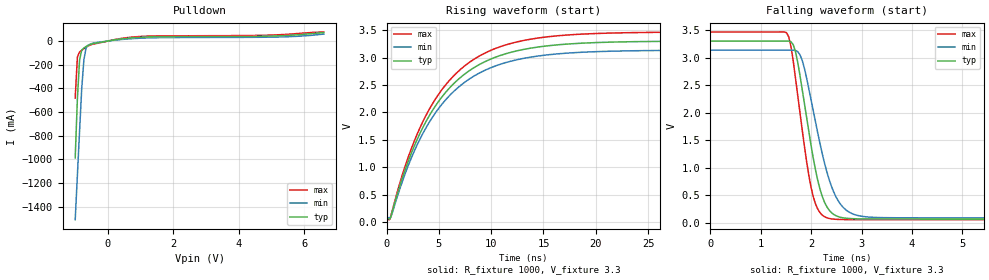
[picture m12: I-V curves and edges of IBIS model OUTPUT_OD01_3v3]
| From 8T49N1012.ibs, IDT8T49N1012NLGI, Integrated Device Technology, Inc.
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| 4.00000e+00   -1.40232e-02   -4.76240e-01   -2.57124e-03
| 4.10000e+00   -3.15805e-02   -7.57960e-01   -1.15576e-02
| 4.20000e+00   -2.28086e-01   -1.04031e+00   -2.65883e-02
| 4.30000e+00   -6.05610e-01   -1.32309e+00   -4.22837e-02
| 4.40000e+00   -9.83731e-01   -1.60621e+00   -8.93892e-02
| 4.50000e+00   -1.36238e+00   -1.88966e+00   -5.31530e-01
| 4.60000e+00   -1.74151e+00   -2.17340e+00   -1.01600e+00
| 4.70000e+00   -2.12106e+00   -2.45742e+00   -1.50101e+00
| 4.80000e+00   -2.50099e+00   -2.74170e+00   -1.98646e+00
| 4.90000e+00   -2.88126e+00   -3.02624e+00   -2.47229e+00
| 5.00000e+00   -3.26181e+00   -3.31101e+00   -2.95842e+00
| 5.10000e+00   -3.64262e+00   -3.59599e+00   -3.44478e+00
| 5.20000e+00   -4.02364e+00   -3.88118e+00   -3.93135e+00
| 5.30000e+00   -4.40484e+00   -4.16656e+00   -4.41808e+00
| 5.40000e+00   -4.78621e+00   -4.45212e+00   -4.90496e+00
| 5.50000e+00   -5.16771e+00   -4.73783e+00   -5.39197e+00
| 5.60000e+00   -5.54933e+00   -5.02369e+00   -5.87906e+00
| 5.70000e+00   -5.93104e+00   -5.30969e+00   -6.36623e+00
| 5.80000e+00   -6.31284e+00   -5.59582e+00   -6.85344e+00
| 5.90000e+00   -6.69471e+00   -5.88206e+00   -7.34069e+00
| 6.00000e+00   -7.07663e+00   -6.16842e+00   -7.82796e+00
| 6.10000e+00   -7.45860e+00   -6.45487e+00   -8.31524e+00
| 6.20000e+00   -7.84061e+00   -6.74142e+00   -8.80252e+00
| 6.30000e+00   -8.22265e+00   -7.02805e+00   -9.28980e+00
| 6.40000e+00   -8.60472e+00   -7.31476e+00   -9.77706e+00
| 6.50000e+00   -8.98680e+00   -7.60155e+00   -1.02643e+01
| 6.60000e+00   -9.36890e+00   -7.88842e+00   -1.07515e+01
[Model] OUTPUT_OD01_3v3
Model_type   Open_drain
Polarity   Non-Inverting
|   typ   min   max
C_comp   2pF   1.5pF   2.5pF
Vmeas = 1.65V
Rref = 1000
Cref = 0
Vref = 3.3V
|   typ   min   max
[Voltage range]   3.3V   3.135V   3.465V
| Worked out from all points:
|   slope of the pulldown table from 0 to 0.495 V, typ, clamps not added: 24.6 ohm
|   rising waveform, R_fixture 1000, V_fixture 3.3: 20-80 % time 5.81ns typ, 5.87ns min, 5.76ns max; typ from 0.066 V to 3.3 V
|   falling waveform, R_fixture 1000, V_fixture 3.3: 20-80 % time 364ps typ, 455ps min, 312ps max; typ from 3.3 V to 0.066 V
[Pulldown]
|Note, modeling breaks down at 250mA and above.  This is well beyond the functional   |
|operating range of the device.  Should this scenario occur, catastrophic failure and   |
|possible damage to the device and/or board is of higher concern than the I-V curve   |
|behavior.  The IBIS checker will flag currents in excess of 10A with warnings.  Lines   |
|with currents in excess of 0.35 A have been commented out.  The points still remain|
|available to the user if the user desires to use them.   |
|Voltage   I (typ)   I (min)   I (max)
|-3.30000e+00   -1.82727e+01   -1.44945e+01   -2.25188e+01
|-2.84000e+00   -1.48135e+01   -1.18930e+01   -1.81101e+01
|-2.38000e+00   -1.13544e+01   -9.29315e+00   -1.37009e+01
|-1.92000e+00   -7.89630e+00   -6.69545e+00   -9.29169e+00
|-1.46000e+00   -4.44012e+00   -4.10091e+00   -4.88327e+00
-1V       -988.4mA   -1.511A    -482.7mA
-932.9mV  -486.9mA   -1.134A    -135.3mA
-866.8mV  -160.7mA   -762.8mA   -91.83mA
-800.8mV  -75.99mA   -401.8mA   -79.06mA
-734.7mV  -58.48mA   -159.9mA   -65.71mA
-668.6mV  -46.68mA   -58.37mA   -52.4mA
-602.5mV  -36.75mA   -35.1mA    -41.15mA
-272.1mV  -13.27mA   -9.902mA   -16.62mA
388.7mV   16.58mA    12.16mA    20.94mA
983.4mV   31.27mA    23.72mA    38.36mA
5.121V    42.77mA    33.37mA    51.42mA
6.6V      70.77mA    58.76mA    76.56mA
[Ramp]
|   typ   min   max
dV/dt_r   1.942/5.814n   1.829/5.871n   2.048/5.757n
dV/dt_f   1.94/0.364n   1.829/0.455n   2.047/0.311n
R_load =   50.0000
[Rising Waveform]
R_fixture = 1000
V_fixture = 3.3
V_fixture_min = 3.135
V_fixture_max = 3.465
C_fixture = 0.0p
| Time   typ   min   max
0s        65.94mV    87.06mV    53.89mV
444.4ps   124.6mV    112.5mV    142.9mV
1.511ns   806.8mV    744.9mV    866.2mV
2.622ns   1.376V     1.285V     1.466V
4.444ns   2.053V     1.93V      2.175V
6.844ns   2.601V     2.455V     2.746V
9.822ns   2.961V     2.803V     3.118V
13.2ns    3.151V     2.988V     3.314V
17.91ns   3.253V     3.088V     3.418V
40ns      3.3V       3.135V     3.465V
[Falling Waveform]
R_fixture = 1000
V_fixture = 3.3
V_fixture_min = 3.135
V_fixture_max = 3.465
C_fixture = 0.0p
| Time   typ   min   max
0s        3.3V       3.135V     3.465V
1.511ns   3.301V     3.135V     3.453V
1.689ns   3.112V     3.13V      2.635V
1.822ns   2.422V     2.951V     1.69V
2.044ns   1.16V      2.02V      463.6mV
2.222ns   471.4mV    1.246V     135.3mV
2.444ns   151.5mV    563.3mV    63.82mV
2.8ns     72.74mV    168.8mV    54.84mV
3.467ns   66.45mV    90.34mV    54.13mV
40ns      65.94mV    87.07mV    53.89mV
